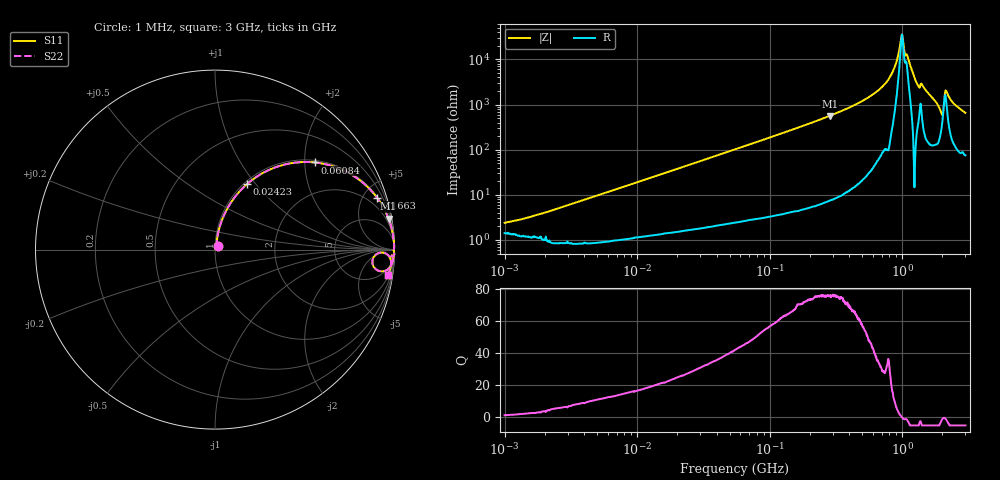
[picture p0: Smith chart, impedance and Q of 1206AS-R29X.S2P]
!s-Parameter Generated by FASTRON Sdn. Bhd.
!FASTRON P/N : 1206AS-R29X
!Keysight Technologies: E4991B_MY54100416_A.01.15
!Date created: Thu Nov 16 10:56:45 2023
!Version  : Rev00 Thu Nov 16 10:56:45 2023
!Data & Calibration Information:
!Freq	S11	S21	S12	S22
!PortZ  Port1:50+j0  Port2:50+j0
!When reading reference impedance value at option line is always used.
! Remarks : This data is being provided solely for informational purposes.
# Hz S dB R 50
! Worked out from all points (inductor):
!   1601 points, 1 MHz to 3 GHz, reference 50 ohm
!   read as one part in series: L = 309 nH near 1.76 MHz
!   highest Q = 75.7 at 284.1 MHz (marker M1), where L = 315 nH
!   self-resonance near 997.7 MHz
!   S11 on the Smith chart (normalised r, x): 1 MHz: 1.03, +0.04; 24.23 MHz: 1.03, +0.91; 60.84 MHz: 1.05, +2.26; 166.3 MHz: 1.09, +6.26; 3 GHz: 3, -13
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1000000  -32.48 52.9  -0.12 -1.1  -0.12 -1.1  -32.48 52.9
3804036  -22.71 79.4  -0.09 -4.2  -0.09 -4.2  -22.71 79.4
1.447069e7  -11.69 72.2  -0.42 -15.1  -0.42 -15.1  -11.69 72.2
2.422863e7  -7.80 63.9  -0.93 -24.0  -0.93 -24.0  -7.80 63.9
5.477226e7  -3.04 43.9  -3.18 -44.8  -3.18 -44.8  -3.04 43.9
6.084121e7  -2.61 41.0  -3.66 -47.7  -3.66 -47.7  -2.61 41.0
1.663456e8  -0.46 17.6  -10.37 -71.5  -10.37 -71.5  -0.46 17.6
2.083556e8  -0.29 14.1  -12.28 -75.2  -12.28 -75.2  -0.29 14.1
2.841474e8  -0.16 10.1  -15.15 -79.2  -15.15 -79.2  -0.16 10.1
5.528145e8  -0.03 4.0  -23.09 -84.8  -23.09 -84.8  -0.03 4.0
6.889699e8  -0.02 2.5  -27.25 -85.7  -27.25 -85.7  -0.02 2.5
7.925923e8  -0.01 1.5  -31.37 -86.8  -31.37 -86.8  -0.01 1.5
8.848309e8  -0.01 0.8  -37.13 -82.6  -37.13 -82.6  -0.01 0.8
9.682285e8  -0.02 0.2  -46.92 -55.1  -46.92 -55.1  -0.02 0.2
9.977393e8  -0.02 0.0  -51.05 -2.2  -51.05 -2.2  -0.02 0.0
1.313842e9  -0.05 -2.1  -28.64 80.5  -28.64 80.5  -0.05 -2.1
1.437675e9  -0.05 -2.2  -28.10 80.4  -28.10 80.4  -0.05 -2.2
1.960646e9  -0.50 -7.4  -17.28 62.1  -17.28 62.1  -0.50 -7.4
2.000286e9  -0.91 -6.9  -16.41 45.4  -16.41 45.4  -0.91 -6.9
2.177892e9  -0.20 -2.8  -25.54 62.5  -25.54 62.5  -0.20 -2.8
2.455801e9  -0.14 -5.4  -20.53 77.4  -20.53 77.4  -0.14 -5.4
3e9  -0.25 -8.5  -16.56 74.9  -16.56 74.9  -0.25 -8.5
